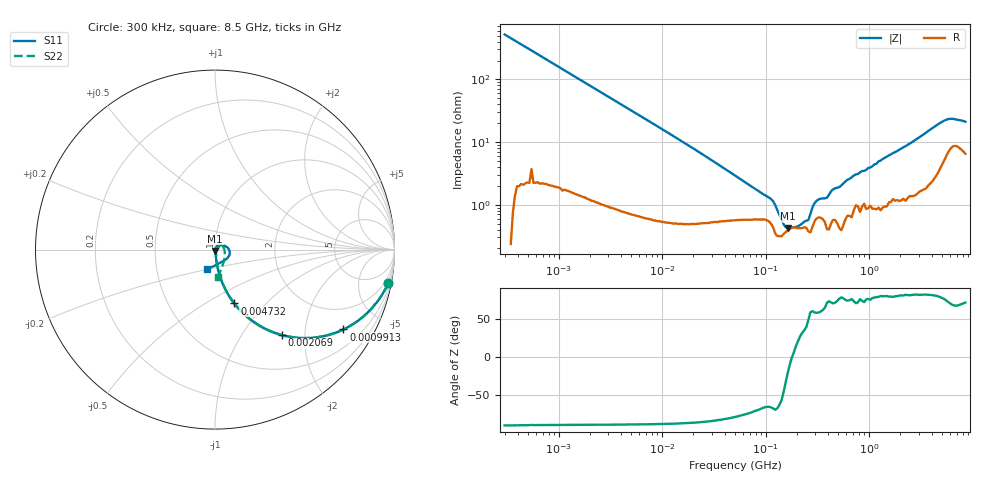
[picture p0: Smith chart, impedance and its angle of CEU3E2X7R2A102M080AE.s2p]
! S-parameter Generated by TDK Corporation
! Copyright(C) 2015 TDK Corporation.
! All Rights Reserved.
! TDK P/N: CEU3E2X7R2A102M080AE (Multilayer Ceramic Chip Capacitors)
! Property: C=1nF
! Size(LxWxT): 1.6x0.8x0.8mm, 0.063x0.031x0.031inches
! Model Type: s2p (Touchstone File Format Version 1.0)
! Frequency: DC=Yes Start=0.3MHz Stop=8500MHz 225points Log-sweep
! Note:
! Model Generated on Jun. 23, 2015
! Hash(MD5):
! Port Assignments:
!  1 ---| |--- 2
! Applicable Conditions:
!  Temperature = 25 degC
!  DC Bias Voltage = 0 V
!  Small Signal Operation
! Terms and conditions regarding TDK Simulation Models
! (1)This simulation model is being provided solely for informational purposes. Please refer to the specifications of the products in terms of detailed characteristics of such products.
! (2)In no event shall TDK Corporation of any of its subsidiaries be liable for any loss or damage arising, directly or indirectly,
!  From any information contained in this simulation model, including, but not limited to loss or damages arising from any inaccuracies, omissions or errors in connection with such information.
! (3)Any and all copyrights on this simulation model are owned by TDK Corporation.
!  Duplication or redistribution of this simulation model without prior written permission from TDK Corporation is prohibited.
! (4)This simulation model is subject to any modification or change without any prior notice.
! (5)Neither TDK Corporation nor any of its subsidiaries shall make any warranty, express or implied,
!  Including but not limited to the correctness, implied warranties of merchantability and fitness for a particular purpose with respect to this simulation models.
! (6)The use of this simulation model shall be deemed to have consented to the terms and conditions hereof.
# MHz S MA R 50
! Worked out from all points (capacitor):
!   224 points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, 300 kHz to 8.5 GHz, reference 50 ohm
!   read as one part in series: C = 1.01 nF near 314.1 kHz
!   lowest |Z| = 418 mohm at 163.1 MHz (marker M1)
!   series resonance near 179.3 MHz, so ESL is about 780 pH
!   S11 on the Smith chart (normalised r, x): 300 kHz: 1, -10; 991.3 kHz: 1.04, -3.19; 2.069 MHz: 1.02, -1.54; 4.732 MHz: 1.01, -0.68; 8.5 GHz: 0.90, -0.19
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0.3  0.9821 -11.0  0.1885 78.9  0.1885 79.0  0.9821 -11.0
0.9913414  0.8426 -31.8  0.5273 57.5  0.5275 57.5  0.8426 -31.9
1.72111  0.6738 -46.8  0.7288 42.4  0.7292 42.4  0.674 -46.8
2.068572  0.6058 -51.8  0.7863 37.3  0.7866 37.3  0.6058 -51.9
4.732045  0.3187 -70.2  0.9407 18.6  0.9411 18.6  0.3188 -70.2
9.430415  0.1669 -78.7  0.9801 9.6  0.9807 9.6  0.1669 -78.6
51.67171  0.02872 -82.6  0.9928 1.5  0.9932 1.5  0.03223 -77.0
163.0757  0.007746 -89.9  0.9939 -0.3  0.9944 -0.3  0.009247 -65.6
246.6485  0.007236 -91.2  0.9915 -0.8  0.9923 -0.8  0.006377 -82.6
283.1228  0.004987 -74.7  0.9922 -1.1  0.9928 -1.1  0.001698 -37.7
324.9909  0.00289 -30.2  0.9908 -1.3  0.9914 -1.3  0.00507 -25.3
408.9767  0.003224 -72.0  0.9924 -1.7  0.9931 -1.7  0.00129 -68.4
514.6664  0.001579 155.5  0.9895 -2.2  0.9901 -2.2  0.003528 -128.5
743.4462  0.006975 -17.1  0.9866 -3.2  0.9874 -3.2  0.008326 39.3
1124.446  0.004791 35.0  0.9879 -4.9  0.9883 -4.9  0.006764 -5.7
1177.346  0.005238 10.8  0.9864 -5.0  0.9871 -5.0  0.001948 4.1
1232.735  0.007617 20.1  0.9877 -5.3  0.9882 -5.3  0.007052 43.2
1290.729  0.005393 41.9  0.9859 -5.6  0.9867 -5.6  0.002222 43.2
1351.452  0.007546 8.9  0.9864 -5.8  0.9871 -5.8  0.007648 67.8
1551.304  0.008817 18.9  0.9842 -6.7  0.9851 -6.7  0.007054 41.6
2240.89  0.006636 37.7  0.9814 -9.5  0.9822 -9.5  0.006798 33.0
8500  0.1161 -112.4  0.9142 -31.9  0.9144 -32.0  0.1519 -83.0
